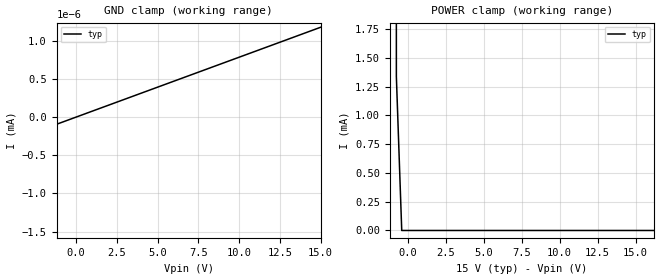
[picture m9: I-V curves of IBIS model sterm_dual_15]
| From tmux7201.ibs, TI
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| sterm_dual_15
[Model]   sterm_dual_15
Model_type   Terminator
|   typ   min   max
C_comp   4.014581e-11   NA   NA
[Voltage Range]   15   NA   NA
[Temperature Range]   27   NA   NA
[Power Clamp Reference]   15   NA   NA
[GND Clamp Reference]   0   NA   NA
[GND Clamp]
|   Voltage   I(typ)   I(min)   I(max)
-20V      -10.37A    NA         NA
-15.4V    -9.306nA   NA         NA
-15.05V   -1.181nA   NA         NA
15V       1.176nA    NA         NA
[POWER Clamp]
|   Voltage   I(typ)   I(min)   I(max)
-5V       13.27A     NA         NA
-1.111V   275.7mA    NA         NA
-757.6mV  1.337mA    NA         NA
-404mV    6.544nA    NA         NA
30V       -1.177nA   NA         NA
